[IBIS Ver]  4.0
[File Name]  lpc3180_01_lfbga320.ibs
[File Rev]  1.0
[Date]  Fri Aug 18 10:34:29 2006
[Source]  Package model from Ansoft Q3D Extractor 7.1.1
[Notes]   IO models Rev 0.20 IBIS Model Design Automation Generation
[Copyright]  NXP Semiconductors 2006,2007. All rights reserved.
|   LPC3180_01_LFBGA320 (320 LFBGA package) IBIS Model
[Disclaimer]
| NXP Semiconductors warrants and represents that the IBIS models
| identified herein are owned by NXP Semiconductors (NXP).  The
| models provided are not warranted as fully representing all of the
| operating characteristics and specifications of the semiconductor
| products to which the models relate.  Moreover, unless there is a
| signed, written agreement to the contrary, these models are furnished
| on an "as is" basis without support or warranty of any kind, either
| expressed or implied, regarding the use thereof, and NXP
| specifically disclaims all implied warranties of merchantability and
| fitness of the models for any purpose.
| NXP does not assume any liability arising out of the application
| or use of these IBIS models including infringement of patents and
| copyrights, nor does NXP convey any license under its patents and
| copyrights or the rights of others.
| NXP provides IBIS models as a service to our customers.  You and
| your company shall not distribute, convey, sell, or give these models
| to anyone else without receiving prior written permission from
| NXP.
[Define Package Model]  LFBGA320
[Manufacturer]  NXP Semiconductors
[OEM]  NXP Semiconductors
[Description] IBIS model for the LPC3180/01
| Full package IBIS model.
| Model includes all substrate features e.g.
| vias, bondwires, metal interconnect,
| dielectrics and mold compound.
| AC simulation frequency:  100 MHz
[Number Of Pins]  213
[Pin Numbers]
|Pin Num   Terminal Name
AC3   | U1:12STX_CLK1:11
AC2   | U1:12STX_SDA1:12
AC4   | U1:12STX_WS1:10
C24   | U1:ADIN0:181
E22   | U1:ADIN1:180
D23   | U1:ADIN2:182
D3   | U1:DBGEN:97
AD22   | U1:EMC_A[00]:288
AB20   | U1:EMC_A[01]:287
AD23   | U1:EMC_A[02]:286
AD24   | U1:EMC_A[03]:282
AC22   | U1:EMC_A[04]:279
AA21   | U1:EMC_A[05]:278
AC23   | U1:EMC_A[06]:275
AB22   | U1:EMC_A[07]:274
AB23   | U1:EMC_A[08]:271
AA23   | U1:EMC_A[09]:268
Y22   | U1:EMC_A[10]:267
AB24   | U1:EMC_A[11]:266
Y23   | U1:EMC_A[12]:265
AA24   | U1:EMC_A[13]:264
W21   | U1:EMC_A[14]:263
V23   | U1:EMC_CAS_N:255
U24   | U1:EMC_CKE0:248
U23   | U1:EMC_CLK:250
T21   | U1:EMC_CLKIN:249
Y24   | U1:EMC_DQM[0]:262
W23   | U1:EMC_DQM[1]:259
V21   | U1:EMC_DQM[2]:258
W24   | U1:EMC_DQM[3]:257
V24   | U1:EMC_DYCS0_N:253
T23   | U1:EMC_D[00]:246
T22   | U1:EMC_D[01]:245
T24   | U1:EMC_D[02]:244
R24   | U1:EMC_D[03]:243
P21   | U1:EMC_D[04]:242
R23   | U1:EMC_D[05]:241
P24   | U1:EMC_D[06]:238
N21   | U1:EMC_D[07]:237
P23   | U1:EMC_D[08]:236
N24   | U1:EMC_D[09]:233
M22   | U1:EMC_D[10]:232
N23   | U1:EMC_D[11]:231
M24   | U1:EMC_D[12]:229
L22   | U1:EMC_D[13]:228
M23   | U1:EMC_D[14]:227
L24   | U1:EMC_D[15]:226
L23   | U1:EMC_D[16]:223
L21   | U1:EMC_D[17]:222
K24   | U1:EMC_D[18]:221
H21   | U1:EMC_D[19]:220
J24   | U1:EMC_D[20]:219
H24   | U1:EMC_D[21]:214
K23   | U1:EMC_D[22]:213
H22   | U1:EMC_D[23]:209
G23   | U1:EMC_D[24]:208
J21   | U1:EMC_D[25]:207
H23   | U1:EMC_D[26]:206
G24   | U1:EMC_D[27]:203
F24   | U1:EMC_D[28]:200
F21   | U1:EMC_D[29]:199
E23   | U1:EMC_D[30]:198
E24   | U1:EMC_D[31]:196
U21   | U1:EMC_RAS_N:254
V22   | U1:EMC_WR_N:256
AA16   | U1:FLASH_ALE:320
AC21   | U1:FLASH_CE_N:325
AC15   | U1:FLASH_CLE:328
AD21   | U1:FLASH_IO[00]:306
AD20   | U1:FLASH_IO[01]:307
AC19   | U1:FLASH_IO[02]:308
AC20   | U1:FLASH_IO[03]:309
AB19   | U1:FLASH_IO[04]:311
AD19   | U1:FLASH_IO[05]:312
AC17   | U1:FLASH_IO[06]:313
AD18   | U1:FLASH_IO[07]:314
AC18   | U1:FLASH_RDY:319
AA17   | U1:FLASH_RD_N:327
AD17   | U1:FLASH_WR_N:326
T3   | U1:GPIO_00:48
R1   | U1:GPIO_01:47
U3   | U1:GPIO_02:46
T1   | U1:GPIO_03:45
T2   | U1:GPIO_04:42
R2   | U1:GPIO_05:41
H1   | U1:GPI_00:76
K3   | U1:GPI_01:75
J3   | U1:GPI_02:74
AA11   | U1:GPI_03:330
K4   | U1:GPI_04:73
A12   | U1:GPI_05:142
AA3   | U1:GPI_06:24
J1   | U1:GPI_07:72
K2   | U1:GPI_08:69
L2   | U1:GPI_09:68
K1   | U1:GPI_10:67
D10   | U1:GPI_11:141
AB9   | U1:GPO_00:337
AC9   | U1:GPO_01:336
L4   | U1:GPO_02:66
L1   | U1:GPO_03:65
Y3   | U1:GPO_04:26
AB10   | U1:GPO_05:335
M4   | U1:GPO_06:64
M3   | U1:GPO_07:63
M1   | U1:GPO_08:60
N4   | U1:GPO_09:59
M2   | U1:GPO_10:58
AB1   | U1:GPO_11:25
P3   | U1:GPO_12:57
N1   | U1:GPO_13:56
AD9   | U1:GPO_14:334
R4   | U1:GPO_15:55
N2   | U1:GPO_16:54
B12   | U1:GPO_17:140
P1   | U1:GPO_18:51
AC10   | U1:GPO_19:333
AD10   | U1:GPO_20:331
P4   | U1:GPO_21:50
P2   | U1:GPO_22:49
A11   | U1:GPO_23:135
A3   | U1:HIGHCORE:107
Y4   | U1:I2C1_SCL:20
AC1   | U1:I2C1_SDA:21
AD8   | U1:I2C2_SCL:338
AA9   | U1:I2C2_SDA:339
D7   | U1:JTAG_NTRST:113
A6   | U1:JTAG_RTCK:114
B5   | U1:JTAG_TCK:112
B6   | U1:JTAG_TDI:111
A4   | U1:JTAG_TDO:109
A5   | U1:JTAG_TMS:110
D2   | U1:KEY_COL0:90
F4   | U1:KEY_COL1:91
C1   | U1:KEY_COL2:92
C2   | U1:KEY_COL3:94
E4   | U1:KEY_COL4:95
B1   | U1:KEY_COL5:96
G3   | U1:KEY_ROW0:82
F2   | U1:KEY_ROW1:83
E1   | U1:KEY_ROW2:86
F3   | U1:KEY_ROW3:87
D1   | U1:KEY_ROW4:88
E2   | U1:KEY_ROW5:89
Y1   | U1:MS_BS:28
W2   | U1:MS_DIO0:32
U2   | U1:MS_DIO1:31
Y2   | U1:MS_DIO2:30
V4   | U1:MS_DIO3:29
AA1   | U1:MS_SCLK:27
D12   | U1:ONSW:146
C21   | U1:PLL397_LOOP:173
J2   | U1:PWM_OUT1:77
H3   | U1:PWM_OUT2:78
D13   | U1:RESET_N:147
AB12   | U1:RESOUT_N:329
A14   | U1:RTCX_IN:152
A13   | U1:RTCX_OUT:151
W3   | U1:SPI1_CLK:33
V1   | U1:SPI1_DATIN:37
W1   | U1:SPI1_DATIO:34
V3   | U1:SPI2_CLK:38
T4   | U1:SPI2_DATIN:40
V2   | U1:SPI2_DATIO:39
C5   | U1:SYSCLKEN:108
A23   | U1:SYSX_IN:169
B23   | U1:SYSX_OUT:170
AB3   | U1:TST_CLK2:13
B9   | U1:U1_RX:121
B10   | U1:U1_TX:122
B8   | U1:U2_HCTS:117
C7   | U1:U2_RX:118
D9   | U1:U2_TX:120
C6   | U1:U3_RX:115
A7   | U1:U3_TX:116
A2   | U1:U5_RX:105
C4   | U1:U5_TX:106
A1   | U1:U6_IRRX:103
D5   | U1:U6_IRTX:104
B2   | U1:U7_HCTS:98
C3   | U1:U7_RX:99
B3   | U1:U7_TX:100
AA7   | U1:USB_ATX_INT_N:7
AA8   | U1:USB_DAT_VP:3
AC8   | U1:USB_I2C_SCL:340
AD7   | U1:USB_I2C_SDA:2
AD6   | U1:USB_OE_TP_N:6
AB7   | U1:USB_SE0_VM:5
E21   | U1:VDD_AD:178
C10   | U1:VDD_COREFXD12:139
B14   | U1:VDD_FUSE:154
B4   | U1:VDD_IOA:124
AA4   | U1:VDD_IOB:16
AC7   | U1:VDD_IOC:4
U4   | U1:VDD_IOD:36
D20   | U1:VDD_OSC12:168
C22   | U1:VDD_PLL397_12:172
A22   | U1:VDD_PLLHCLK_12:162
B22   | U1:VDD_PLLUSB_12:164
C12   | U1:VDD_RTC12:148
C11   | U1:VDD_RTCCORE12:143
C14   | U1:VDD_RTCOSC12:153
D22   | U1:VSS_AD:176
A10   | U1:VSS_IOA:128
AB5   | U1:VSS_IOB:9
AB8   | U1:VSS_IOC:1
D4   | U1:VSS_IOD:102
B21   | U1:VSS_OSC:171
C23   | U1:VSS_PLL397:174
D19   | U1:VSS_PLLHCLK:161
B20   | U1:VSS_PLLUSB:163
B13   | U1:VSS_RTCCORE:144
C13   | U1:VSS_RTCOSC:150
[Model Data]
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[End Model Data]
[End Package Model]
[Component]   LPC3180_01_LFBGA320
[Manufacturer]  NXP
[Package]
|   typ   min   max
R_pkg   0   0   0  |Values included in package model
L_pkg   0   0   0  |Values included in package model
C_pkg   0   0   0  |Values included in package model
[Package Model]  LFBGA320
| (Pin and IO model definitions)
| IMPORTANT NOTES:
| This model is valid for the following part types:
| LPC3180
| LPC3180/01
| Signal names may be slightly different from the data
| sheet due to the 20 Char length limitation
[Pin]   signal_name   model_name   | comments
C24   ADIN0   NC   |apio3v3 Not Modeled
E22   ADIN1   NC   |apio3v3 Not Modeled
D23   ADIN2   NC   |apio3v3 Not Modeled
D3   DBGEN   bspts3chp
AD22   EMC_A[00]/P1.0   mem1bsptz40pchp
AB20   EMC_A[01]/P1.1   mem1bsptz40pchp
AD23   EMC_A[02]/P1.2   mem1bsptz40pchp
AD24   EMC_A[03]/P1.3   mem1bsptz40pchp
AC22   EMC_A[04]/P1.4   mem1bsptz40pchp
AA21   EMC_A[05]/P1.5   mem1bsptz40pchp
AC23   EMC_A[06]/P1.6   mem1bsptz40pchp
AB22   EMC_A[07]/P1.7   mem1bsptz40pchp
AB23   EMC_A[08]/P1.8   mem1bsptz40pchp
AA23   EMC_A[09]/P1.9   mem1bsptz40pchp
Y22   EMC_A[10]/P1.10   mem1bsptz40pchp
AB24   EMC_A[11]/P1.11   mem1bsptz40pchp
Y23   EMC_A[12]/P1.12   mem1bsptz40pchp
AA24   EMC_A[13]/P1.13   mem1bsptz40pchp
W21   EMC_A[14]/P1.14   mem1bsptz40pchp
AD16   EMC_A[15]/P1.15   mem1bsptz40pchp
AB16   EMC_A[16]/P1.16   mem1bsptz40pchp
AA14   EMC_A[17]/P1.17   mem1bsptz40pchp
AC14   EMC_A[18]/P1.18   mem1bsptz40pchp
AB15   EMC_A[19]/P1.19   mem1bsptz40pchp
AD14   EMC_A[20]/P1.20   mem1bsptz40pchp
AC13   EMC_A[21]/P1.21   mem1bsptz40pchp
AB14   EMC_A[22]/P1.22   mem1bsptz40pchp
AD13   EMC_A[23]/P1.23   mem1bsptz40pchp
A19   EMC_BLS[0]   mem1bsptz40pchp
A17   EMC_BLS[1]   mem1bsptz40pchp
A16   EMC_BLS[2]   mem1bsptz40pchp
D14   EMC_BLS[3]   mem1bsptz40pchp
V23   EMC_CAS_N   mem1bsptz40pchp
U24   EMC_CKE0   mem1bsptz40pchp
AA18   EMC_CKE1   mem1bsptz40pchp
U23   EMC_CLK   mem1bsptz40pchp
T21   EMC_CLKIN   mem1bsptz40pchp
C18   EMC_CS0_N   mem1bsptz40pchp
B18   EMC_CS1_N   mem1bsptz40pchp
B17   EMC_CS2_N   mem1bsptz40pchp
A18   EMC_CS3_N   mem1bsptz40pchp
T23   EMC_D[00]   mem1bsptz40pchp
T22   EMC_D[01]   mem1bsptz40pchp
T24   EMC_D[02]   mem1bsptz40pchp
R24   EMC_D[03]   mem1bsptz40pchp
P21   EMC_D[04]   mem1bsptz40pchp
R23   EMC_D[05]   mem1bsptz40pchp
P24   EMC_D[06]   mem1bsptz40pchp
N21   EMC_D[07]   mem1bsptz40pchp
P23   EMC_D[08]   mem1bsptz40pchp
N24   EMC_D[09]   mem1bsptz40pchp
M22   EMC_D[10]   mem1bsptz40pchp
N23   EMC_D[11]   mem1bsptz40pchp
M24   EMC_D[12]   mem1bsptz40pchp
L22   EMC_D[13]   mem1bsptz40pchp
M23   EMC_D[14]   mem1bsptz40pchp
L24   EMC_D[15]   mem1bsptz40pchp
L23   EMC_D[16]/DDR_DQS0   mem1bsptz40pchp
L21   EMC_D[17]/DDR_DQS1   mem1bsptz40pchp
K24   EMC_D[18]/DDR_NCLK   mem1bsptz40pchp
H21   EMC_D[19]   mem1bsptz40pchp
J24   EMC_D[20]   mem1bsptz40pchp
H24   EMC_D[21]   mem1bsptz40pchp
K23   EMC_D[22]   mem1bsptz40pchp
H22   EMC_D[23]   mem1bsptz40pchp
G23   EMC_D[24]   mem1bsptz40pchp
J21   EMC_D[25]   mem1bsptz40pchp
H23   EMC_D[26]   mem1bsptz40pchp
G24   EMC_D[27]   mem1bsptz40pchp
F24   EMC_D[28]   mem1bsptz40pchp
F21   EMC_D[29]   mem1bsptz40pchp
E23   EMC_D[30]   mem1bsptz40pchp
E24   EMC_D[31]   mem1bsptz40pchp
Y24   EMC_DQM[0]   mem1bsptz40pchp
W23   EMC_DQM[1]   mem1bsptz40pchp
V21   EMC_DQM[2]   mem1bsptz40pchp
W24   EMC_DQM[3]   mem1bsptz40pchp
V24   EMC_DYCS0_N   mem1bsptz40pchp
AB13   EMC_DYCS1_N   mem1bsptz40pchp
AA13   EMC_OE_N   mem1bsptz40pchp
U21   EMC_RAS_N   mem1bsptz40pchp
V22   EMC_WR_N   mem1bsptz40pchp
AA16   FLASH_ALE   mem1bsptz40pchp
AC21   FLASH_CE_N   mem1bsptz40pchp
AC15   FLASH_CLE   mem1bsptz40pchp
AD21   FLASH_IO[00]   mem1bsptz40pchp
AD20   FLASH_IO[01]   mem1bsptz40pchp
AC19   FLASH_IO[02]   mem1bsptz40pchp
AC20   FLASH_IO[03]   mem1bsptz40pchp
AB19   FLASH_IO[04]   mem1bsptz40pchp
AD19   FLASH_IO[05]   mem1bsptz40pchp
AC17   FLASH_IO[06]   mem1bsptz40pchp
AD18   FLASH_IO[07]   mem1bsptz40pchp
AA17   FLASH_RD_N   mem1bsptz40pchp
AC18   FLASH_RDY   mem1bsptz40pchp
AD17   FLASH_WR_N   mem1bsptz40pchp
H1   GPI_00/E_RXD2GPI_00  bspts3chp
K3   GPI_01/SERVICE_N   bspts3chp
J3   GPI_02/CAP2.0/E_RXD3 bspts3chp
AA11   GPI_03   bspts3chp
K4   GPI_04/SPI1_BUSY   bspts3chp
A12   GPI_05/U3_DCD   bspts3chp
AA3   GPI_06/CAP/I2SX_SDA1 bspts3chp
J1   GPI_07/PCAP3.0   bspts3chp
K2   GPI_08/KEY_COL6   bspts3chp
L2   GPI_09/KEY_CL7/E_COL bspts3chp
K1   GPI_10/U4_RX   bspts3chp
D10   GPI_11/U3_RI   bspts3chp
T3   GPIO_00   bspts3chp
R1   GPIO_01   bspts3chp
U3   GPIO_02/KY_RW6/E_MDC bspts3chp
T1   GPIO_03/KY_RW7/E_MIO bspts3chp
T2   GPIO_04/SSEL1/L[22]  bspts3chp
R2   GPIO_05/SSEL0   bspts3chp
AB9   GPO_00/TST_CLK1   bspts3cp
AC9   GPO_01   bspts3chp
L4   GPO_02/MAT1.0/L[0]   bspts3chp
L1   GPO_03/LCDVD[1]   bspts3chp
Y3   GPO_04   bspts3chp
AB10   GPO_05   bspts3cp
M4   GPO_06/PWM4.3/L[18]  bspts3chp
M3   GPO_07/LCDVD[2]   bspts3chp
M1   GPO_08/PWM4.2/L[8]   bspts3chp
N4   GPO_09/PWM4.1/L[9]   bspts3chp
M2   GPO_10/PWM3.6/LCDPWR bspts3chp
AB1   GPO_11   bspts3chp
P3   GPO_12/PWM3.5/LCDLE  bspts3chp
N1   GPO_13/PWM3.4/LCLK   bspts3chp
AD9   GPO_14   bspts3chp
R4   GPO_15/PWM3.3/LCDFP  bspts3chp
N2   GPO_16/PWM3.2/LENAB  bspts3chp
B12   GPO_17   bspts3chp
P1   GPO_18/PWM3.1/LCDLP  bspts3chp
AC10   GPO_19   bspts3chp
AD10   GPO_20   bspts3cp
P4   GPO_21/U4_TX/L[3]   bspts3chp
P2   GPO_22/U7_HRTS/L[14] bspts3cp
A11   GPO_23/HRTS/RTS   bspts3cp
A3   HIGHCORE/LCDVD[17]   bspts3cp
Y4   I2C1_SCL   iic3m4sclt5v_400k
AC1   I2C1_SDA   iic3m4sdat5v_400k
AD8   I2C2_SCL   iic3m4sclt5v_400k
AA9   I2C2_SDA   iic3m4sdat5v_400k
AC3   I2STX_CLK1/MAT3.0   bspts3chp
AC2   I2STX_SDA1/MAT3.1   bspts3chp
AC4   I2STX_WS1/CAP3.0   bspts3chp
D7   JTAG_NTRST   bspts3chp
A6   JTAG_RTCK   bspts1cp
B5   JTAG_TCK   bspts3cp
B6   JTAG_TDI   bspts3cp
A4   JTAG_TDO   bspts1cp
A5   JTAG_TMS   bspts3cp
D2   KEY_COL0/E_TX_CLK   bspts3chp
F4   KEY_COL1/E_RX_CLK   bspts3chp
C1   KEY_COL2/ET_RX_ER   bspts3chp
C2   KEY_COL3/ENET_CRS   bspts3chp
E4   KEY_COL4/ENET_RXD0   bspts3chp
B1   KEY_COL5/ENET_RXD1   bspts3chp
G3   KEY_ROW0/ENET_TX_ER  bspts3chp
F2   KEY_ROW1/ENET_TXD2   bspts3chp
E1   KEY_ROW2/ENET_TXD3   bspts3chp
F3   KEY_ROW3/ENET_TX_EN  bspts3chp
D1   KEY_ROW4/ENET_TXD0   bspts3chp
E2   KEY_ROW5/ENET_TXD1   bspts3chp
Y1   MS_BS/MAT2.1/PWM3.6  bspts3cp
W2   MS_DIO0/MT0.0/PW3.1  bspts3cp
U2   MS_DIO1/MT0.1/PW3.2  bspts3cp
Y2   MS_DIO2/MT0.2/PW3.3  bspts3cp
V4   MS_DIO3/MT0.3/PW3.4  bspts3cp
AA1   MS_SCLK/MT2.0/PW3.5  bspts3cp
W4   vss   gnd
U1   n.c.   bspts3cp
H4   n.c.   bspts3cp
H2   n.c.   bspts3cp
G2   n.c.   bspts1cp
G1   n.c.   bspts3cp
D17   vssco   gnd
D15   n.c.   NC   |apio3v3 Not Modeled
C17   n.c.   NC   |apio3v3 Not Modeled
C16   vssco   gnd
C15   n.c.   NC   |apio3v3 Not Modeled
B19   n.c.   NC   |apio3v3 Not Modeled
B16   n.c.   NC   |apio3v3 Not Modeled
B15   n.c.   NC   |apio3v3 Not Modeled
AD5   n.c.   bspts3cp
AD4   vdde3v3   power
AD3   n.c.   bspts3cp
AC6   n.c.   bspts3cp
AC5   n.c.   bspts3cp
AC12   vdd   power
AC11   n.c.   bspts3chp
AA6   n.c.   bspts3cp
A21   n.c.   NC   |apio3v3 Not Modeled
A20   vssco   power
A15   vssco   power
D12   ONSW   bspts3chp1v2v
AB2   P0.0/I2SRX_CLK1   bspts3chp
AD1   P0.1/I2SRX_WS1   bspts3chp
D11   P0.2/I2SX_SDA0/L[4]  bspts3chp
B11   P0.3/I2SX_CLK0/L[5]  bspts3chp
C9   P0.4/I2SRX_WS0/L[6]  bspts3chp
C8   P0.5/I2STX_SD0/L[7]  bspts3chp
A9   P0.6/I2STX_C0/L[12]  bspts3chp
A8   P0.7/I2STX_W0/L[13]  bspts3chp
C21   PLL397_LOOP   NC   |apio3v3 Not Modeled
J2   PWM_OUT1/LCDVD[16]   bspts3cp
H3   PWM_OUT2/LCDVD[19]   bspts3cp
D13   RESET_N   ipchp1v2t1v8v
AB12   RESOUT_N   bspts3cp
A14   RTCX_IN   NC   |apio3v3 Not Modeled
A13   RTCX_OUT   NC   |apio3v3 Not Modeled
W3   SPI1_CLK/SCK0   bspts1cp
V1   SPI1_DATIN/MISO0   bspts3cp
W1   SPI1_DATIO/MOSI0   bspts1cp
V3   SPI2_CLK/SCK1/L[23]  bspts1cp
T4   SPI2_DTN/MSO1/L[21]  bspts3cp
V2   SPI2_DTI/MSI1/L[20]  bspts1cp
C5   SYSCLKEN/LCDVD[15]   bspts3chp
A23   SYSX_IN   NC   |apio3v3 Not Modeled
B23   SYSX_OUT   NC   |apio3v3 Not Modeled
B24   TS_XOUT   NC   |apio3v3 Not Modeled
A24   TS_YOUT   NC   |apio3v3 Not Modeled
AB3   TST_CLK2   bspts1cp
B9   U1_RX/CAP1.0   bspts3chp
B10   U1_TX   bspts3cp
B8   U2_HCTS/U3_CTS   bspts3cp
C7   U2_RX/U3_DSR   bspts3cp
D9   U2_TX/U3_DTR   bspts3cp
C6   U3_RX   bspts3cp
A7   U3_TX   bspts3cp
A2   U5_RX   bspts3cp
C4   U5_TX   bspts3cp
A1   U6_IRRX   bspts3cp
D5   U6_IRTX   bspts3cp
B2   U7_HCTS/CAP0.1/LIN   bspts3cp
C3   U7_RX/CAP0.0/L[10]   bspts3cp
B3   U7_TX/MT1.1/LC[11]   bspts3cp
AA7   USB_ATX_INT_N   bspts3cp
AA8   USB_DAT_VP/U5_RX   bspts3cp
AC8   USB_I2C_SCL   iic3m4sclt5v_400k
AD7   USB_I2C_SDA   iic3m4sdat5v_400k
AD6   USB_OE_TP_N   bspts3chp
AB7   USB_SE0_VM/U5_TX   bspts3cp
E21   VDD_AD   power
D24   VDD_AD   power
L3   VDD_CORE12   power
K21   VDD_CORE12   power
D6   VDD_CORE12   power
AB6   VDD_CORE12   power
AB18   VDD_CORE12   power
AA2   VDD_CORE12   power
AA12   VDD_CORE12   power
D18   VDD_COREFXD12   power
C10   VDD_COREFXD12   power
Y21   VDD_EMC   power
U22   VDD_EMC   power
P22   VDD_EMC   power
K22   VDD_EMC   power
J22   VDD_EMC   power
G21   VDD_EMC   power
F22   VDD_EMC   power
D21   VDD_EMC   power
AD12   VDD_EMC   power
AC24   VDD_EMC   power
AA20   VDD_EMC   power
B14   VDD_FUSE   power
B7   VDD_IOA   power
B4   VDD_IOA   power
AA4   VDD_IOB   power
AC7   VDD_IOC   power
AB11   VDD_IOC   power
AA19   VDD_IOC   power
AA15   VDD_IOC   power
U4   VDD_IOD   power
G4   VDD_IOD   power
D20   VDD_OSC12   NC   |apio3v3 Not Modeled
C22   VDD_PLL397_12   NC   |apio3v3 Not Modeled
A22   VDD_PLLHCLK_12   NC   |apio3v3 Not Modeled
B22   VDD_PLLUSB_12   NC   |apio3v3 Not Modeled
C12   VDD_RTC12   power
C11   VDD_RTCCORE12   power
C14   VDD_RTCOSC12   NC   |apio3v3 Not Modeled
D22   VSS_AD   power
R3   VSS_CORE   power
R21   VSS_CORE   power
J4   VSS_CORE   power
D8   VSS_CORE   power
D16   VSS_CORE   power
C20   VSS_CORE   power
AB17   VSS_CORE   power
AA5   VSS_CORE   power
AA10   VSS_CORE   power
W22   VSS_EMC   power
R22   VSS_EMC   power
N22   VSS_EMC   power
M21   VSS_EMC   power
J23   VSS_EMC   power
G22   VSS_EMC   power
F23   VSS_EMC   power
C19   VSS_EMC   power
AD11   VSS_EMC   power
AB21   VSS_EMC   power
AA22   VSS_EMC   power
A10   VSS_IOA   power
AB5   VSS_IOB   power
AD15   VSS_IOC   power
AC16   VSS_IOC   power
AB8   VSS_IOC   power
N3   VSS_IOD   power
F1   VSS_IOD   power
E3   VSS_IOD   power
D4   VSS_IOD   power
B21   VSS_OSC   power
C23   VSS_PLL397   power
D19   VSS_PLLHCLK   power
B20   VSS_PLLUSB   power
B13   VSS_RTCCORE   power
C13   VSS_RTCOSC   power
[Model Selector] ipchp1v2t1v8v
ipchp1v2t1v8v_p   Plain input Mode (p1=0, p2=1)
ipchp1v2t1v8v_pd   Pull Down Mode (p1=1, p2=1)
ipchp1v2t1v8v_pu   Pull Up Mode (p1=0, p2=0)
ipchp1v2t1v8v_r   Repeater Mode (p1=1, p2=0)
[Model Selector] mem1bsptz40pchp
m1bsptz40pchp_p_sh   Plain input Mode (p1=0, p2=1)
m1bsptz40pchp_p_sl   Plain input Mode (p1=0, p2=1)
m1bsptz40pchp_pd_sh   Pull Down Mode (p1=1, p2=1)
m1bsptz40pchp_pd_sl   Pull Down Mode (p1=1, p2=1)
m1bsptz40pchp_pu_sh   Pull Up Mode (p1=0, p2=0)
m1bsptz40pchp_pu_sl   Pull Up Mode (p1=0, p2=0)
m1bsptz40pchp_r_sh   Repeater Mode (p1=1, p2=0)
m1bsptz40pchp_r_sl   Repeater Mode (p1=1, p2=0)
[Model Selector] bspts3chp1v2v
bspts3chp1v2v_p   Plain input Mode (p1=0, p2=1)
bspts3chp1v2v_pd   Pull Down Mode (p1=1, p2=1)
bspts3chp1v2v_pu   Pull Up Mode (p1=0, p2=0)
bspts3chp1v2v_r   Repeater Mode (p1=1, p2=0)
| |   Rev 0.20 IBIS Model Design Automation Generation   |
| |   N O N - S I L I C O N   C O R R E L A T E D   |
| |   This IBIS [Model] is pre-Beta tactical support   |
| |  Note: this IBIS [Model] contains clamp curves generated   |
| |   through simulation which should not be relied upon   |
| E-Mail Support : helpdesk.ltg@philips.com
| WWW Support   : http://pww.ltg.sc.philips.com/cio
| Generated at   : Philips Semiconductors LTG/CIO-Nijmegen
| Workstation   : nyhc02
| Date/Time   : 2004 Nov 4 (Thu) 11:48:34
| Pcc090lp jliolib_p50 3.1
|   0.90 um 3.3V pad library
|   five level metal
|   dual oxide
|   single threshold voltage
|   nominal line mixed supply
|   parasitic extracted netlists
| Process block b5
| bspt16mchp
|   Bidirectional Pad 3v3
|   3state Output
|   Plain Input
|   CMOS
|   Programmable between
|   - (p1=0, p2=1) plain input
|   - (p1=0, p2=0) with Pull Up
|   - (p1=1, p2=1) with Pull Down
|   - (p1=1, p2=0) with Repeater
|   Characterized at Core 1.2V and I/O 3.3V
| Plain input Mode (p1=0, p2=1)
[Model Selector] bspts1cp
bspts1cp_p   Plain input Mode (p1=0, p2=1)
bspts1cp_pd   Pull Down Mode (p1=1, p2=1)
bspts1cp_pu   Pull Up Mode (p1=0, p2=0)
bspts1cp_r   Repeater Mode (p1=1, p2=0)
[Model Selector] bspts3chp
bspts3chp_p   Plain input Mode (p1=0, p2=1)
bspts3chp_pd   Pull Down Mode (p1=1, p2=1)
bspts3chp_pu   Pull Up Mode (p1=0, p2=0)
bspts3chp_r   Repeater Mode (p1=1, p2=0)
[Model Selector] bspts3cp
bspts3cp_p   Plain input Mode (p1=0, p2=1)
bspts3cp_pd   Pull Down Mode (p1=1, p2=1)
bspts3cp_pu   Pull Up Mode (p1=0, p2=0)
bspts3cp_r   Repeater Mode (p1=1, p2=0)
| Models and submodels in the file (30): iic3m4sdat5v_400k (I/O_open_drain), iic3m4sclt5v_400k (I/O_open_drain), ipchp1v2t1v8v_p (Input), ipchp1v2t1v8v_pd (Input), ipchp1v2t1v8v_pu (Input), ipchp1v2t1v8v_r (Input), m1bsptz40pchp_p_sh (I/O), m1bsptz40pchp_p_sl (I/O), m1bsptz40pchp_pd_sh (I/O), m1bsptz40pchp_pd_sl (I/O), m1bsptz40pchp_pu_sh (I/O), m1bsptz40pchp_pu_sl (I/O), m1bsptz40pchp_r_sh (I/O), m1bsptz40pchp_r_sl (I/O), bspts3chp1v2v_p (I/O), bspts3chp1v2v_pd (I/O), bspts3chp1v2v_pu (I/O), bspts3chp1v2v_r (I/O), bspts1cp_p (I/O), bspts1cp_pd (I/O), bspts1cp_pu (I/O), bspts1cp_r (I/O), bspts3chp_p (I/O), bspts3chp_pd (I/O), bspts3chp_pu (I/O), bspts3chp_r (I/O), bspts3cp_p (I/O), bspts3cp_pd (I/O), bspts3cp_pu (I/O), bspts3cp_r (I/O)
